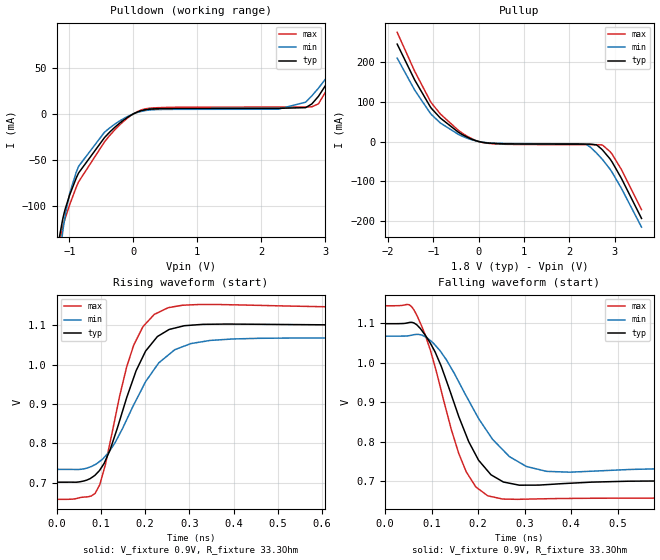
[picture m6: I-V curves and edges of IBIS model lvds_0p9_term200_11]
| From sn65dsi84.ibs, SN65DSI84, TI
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|   Model
[Model]   lvds_0p9_term200_11
Model_type   Output
Polarity   Non-Inverting
Vmeas = 0.9
Vref = 0.9
Cref = 1pF
Rref = 50
|   typ   min   max
C_comp   0.4797pF   0.3035pF   0.7186pF
[Voltage Range]   1.8   1.65   1.95
[Temperature Range]   27   125   -40
[Pullup Reference]   1.8   1.65   1.95
[Pulldown Reference]   -0   -0   -0
[Power Clamp Reference]   1.8   1.65   1.95
[GND Clamp Reference]   -0   -0   -0
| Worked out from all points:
|   slope of the pulldown table from 0 to 0.27 V, typ, clamps not added: 51.4 ohm
|   slope of the pullup table from 0 to 0.27 V, typ, clamps not added: 61.8 ohm
|   falling waveform, V_fixture 0.9V, R_fixture 33.3Ohm: 20-80 % time 78.1ps typ, 101ps min, 70.7ps max; typ from 1.1 V to 0.701 V
|   rising waveform, V_fixture 0.9V, R_fixture 33.3Ohm: 20-80 % time 74.8ps typ, 96.9ps min, 61.5ps max; typ from 0.702 V to 1.1 V
[Pulldown]
|   Voltage   I(typ)   I(min)   I(max)
-1.8V     -663.5mA   -698.3mA   -654.1mA
-1.152V   -133mA     -155.2mA   -138.3mA
-1.103V   -114.8mA   -128.5mA   -123.5mA
-995.4mV  -88.43mA   -86.87mA   -99.1mA
-855mV    -64.32mA   -57.06mA   -74mA
-450mV    -25.77mA   -19.92mA   -30.44mA
-190.8mV  -8.813mA   -6.712mA   -10.55mA
262.8mV   5.211mA    4.296mA    6.247mA
2.261V    6.066mA    5.115mA    7.465mA
2.693V    6.825mA    12.8mA     7.516mA
2.893V    19.13mA    28mA       11.02mA
3.595V    94.35mA    91.7mA     92.44mA
[Pullup]
|   Voltage   I(typ)   I(min)   I(max)
-1.8V     243.6mA    208.6mA    273mA
-1.411V   153.4mA    128.1mA    175.1mA
-1.049V   83.67mA    68.16mA    97.38mA
-450mV    23.31mA    17.93mA    27.99mA
-104.4mV  3.7mA      2.841mA    4.485mA
192.6mV   -3.677mA   -3.117mA   -4.305mA
2.374V    -6.52mA    -7.371mA   -7.98mA
2.606V    -8.841mA   -29.54mA   -8.036mA
2.736V    -21.59mA   -45.56mA   -9.159mA
2.903V    -44.29mA   -69.89mA   -25.95mA
3.141V    -90.33mA   -115.3mA   -68.19mA
3.595V    -192.4mA   -214.2mA   -170.4mA
[Ramp]
R_load = 33.3
|   typ   min   max
dV/dt_r   0.23878/7.4807e-11   0.200243/9.68913e-11   0.29174/6.14966e-11
dV/dt_f   0.238397/7.81385e-11   0.200032/1.00718e-10   0.29169/7.06845e-11
[Falling Waveform]
V_fixture = 0.9V
V_fixture_min = 0.9V
V_fixture_max = 0.9V
R_fixture = 33.3Ohm
C_fixture = 0F
|   Time   V(typ)   V(min)   V(max)
0s        1.099V     1.067V     1.144V
63.2ps    1.1V       1.071V     1.132V
87.21ps   1.069V     1.065V     1.068V
107.7ps   1.027V     1.045V     989.4mV
158.4ps   864.5mV    952mV      771.2mV
195.1ps   767.1mV    872.1mV    686.3mV
220.7ps   726.7mV    824.7mV    663.8mV
267.3ps   695.6mV    762.9mV    655.2mV
347.2ps   692mV      725.5mV    656.3mV
1ns       701.5mV    733.9mV    658mV
[Rising Waveform]
V_fixture = 0.9V
V_fixture_min = 0.9V
V_fixture_max = 0.9V
R_fixture = 33.3Ohm
C_fixture = 0F
|   Time   V(typ)   V(min)   V(max)
0s        701.6mV    734.1mV    658mV
87.21ps   719.5mV    746.3mV    673.1mV
97.64ps   732.1mV    754.5mV    695mV
120.8ps   783.1mV    782.3mV    801.9mV
158.4ps   916mV      860.2mV    994.3mV
174.5ps   967.7mV    898.2mV    1.05V
201.2ps   1.035V     956.9mV    1.104V
252.4ps   1.088V     1.025V     1.145V
397.4ps   1.103V     1.065V     1.152V
1ns       1.1V       1.068V     1.144V
